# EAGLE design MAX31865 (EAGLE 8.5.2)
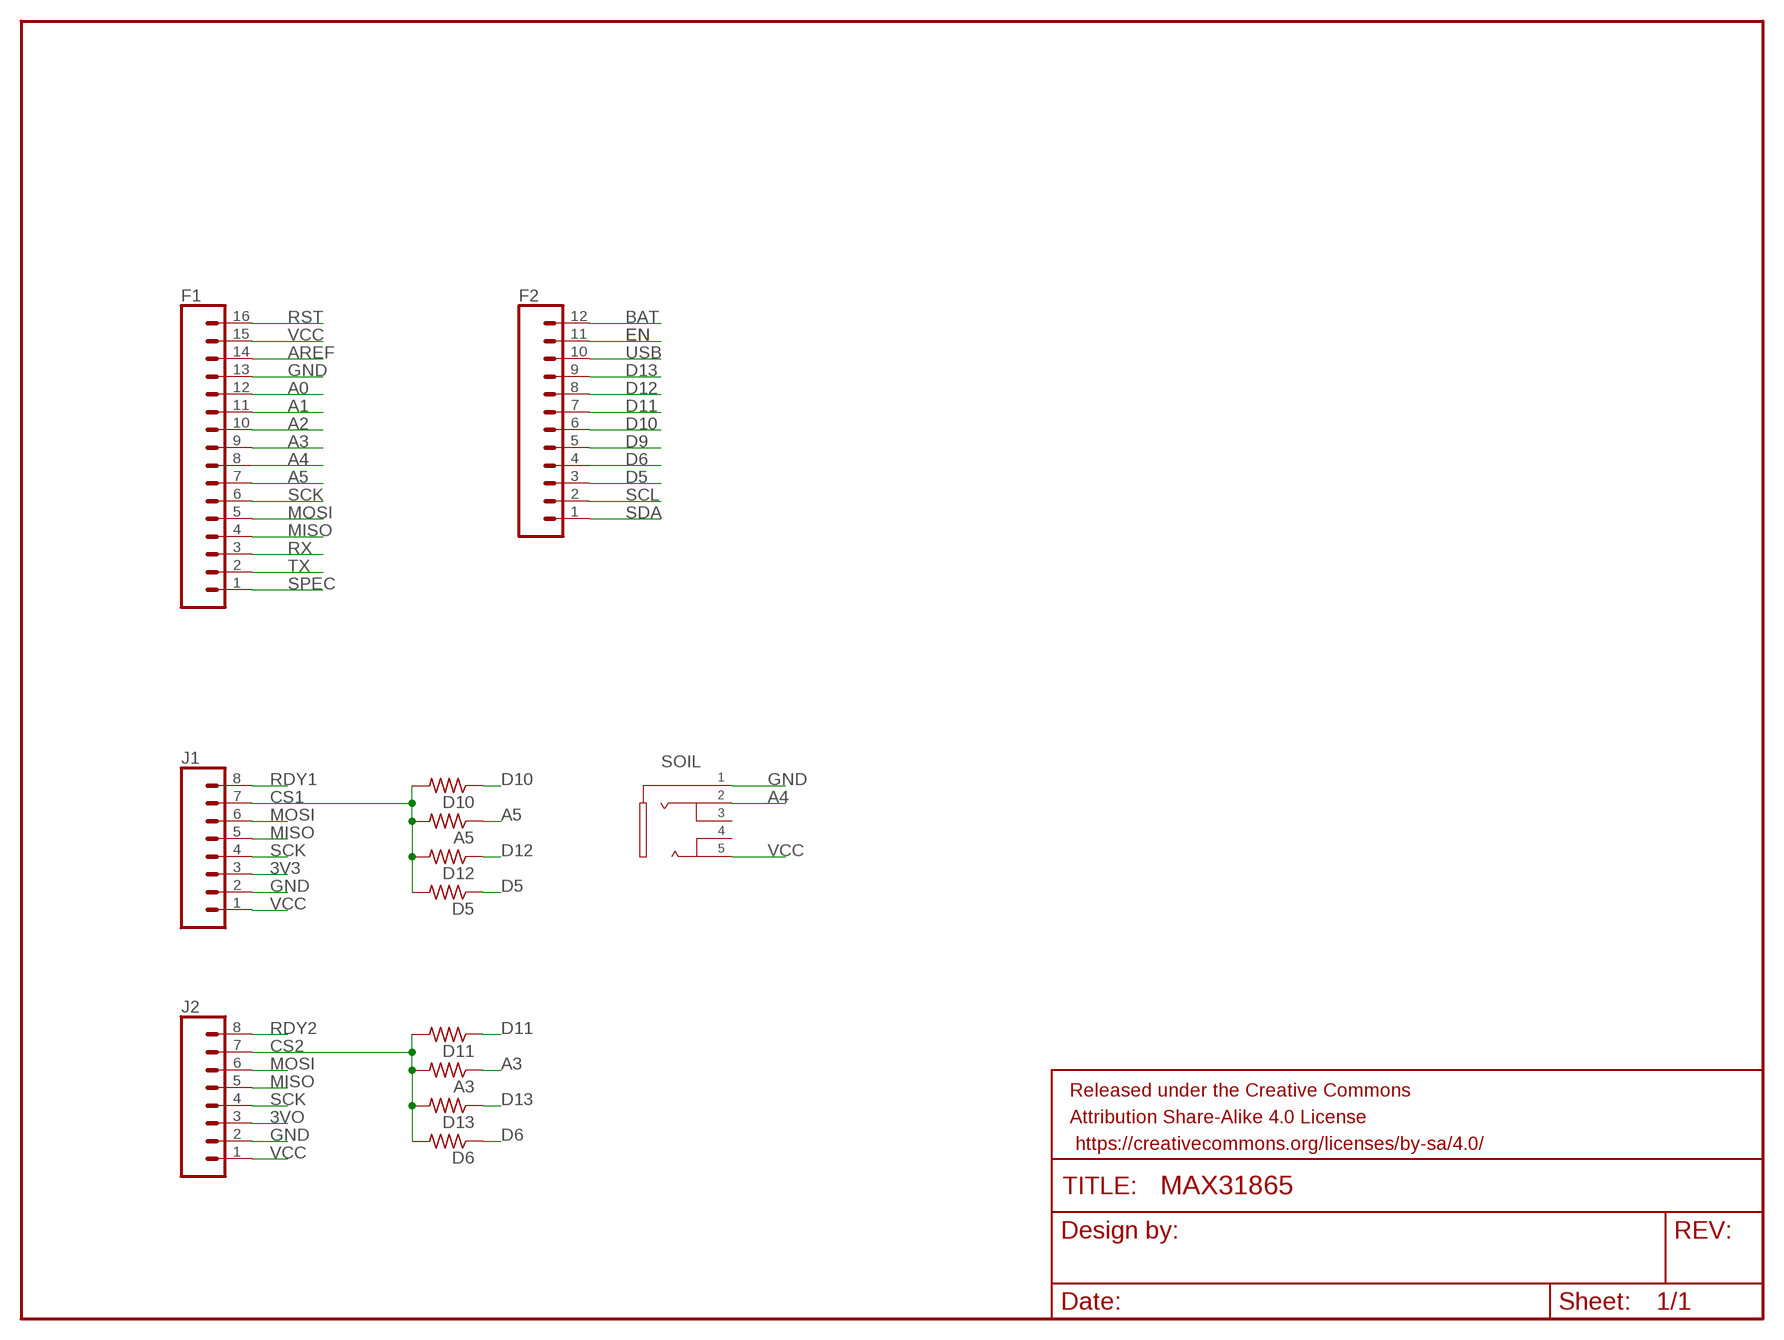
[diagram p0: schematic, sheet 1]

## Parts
A3  R-US_R0603  [R0603]
A5  R-US_R0603  [R0603]
D5  R-US_R0603  [R0603]
D6  R-US_R0603  [R0603]
D10  R-US_R0603  [R0603]
D11  R-US_R0603  [R0603]
D12  R-US_R0603  [R0603]
D13  R-US_R0603  [R0603]
F1  CONN_16  [1X16]
F2  CONN_12  [1X12]
FRAME1  FRAME-LETTER  [CREATIVE_COMMONS]
J1  CONN_08"  [1X08]
J2  CONN_08"  [1X08]
SOIL  JW-PJ-307-5H  [JW-PJ-307-5H]

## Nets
3V3: J1.3
3VO: J2.3
A0: F1.12
A1: F1.11
A2: F1.10
A3: A3.1 F1.9
A4: F1.8 SOIL.2
A5: A5.1 F1.7
AREF: F1.14
BAT: F2.12
CS1: A5.2 D5.2 D10.2 D12.2 J1.7
CS2: A3.2 D6.2 D11.2 D13.2 J2.7
D5: D5.1 F2.3
D6: D6.1 F2.4
D9: F2.5
D10: D10.1 F2.6
D11: D11.1 F2.7
D12: D12.1 F2.8
D13: D13.1 F2.9
EN: F2.11
GND: F1.13 J1.2 J2.2 SOIL.1
MISO: F1.4 J1.5 J2.5
MOSI: F1.5 J1.6 J2.6
RDY1: J1.8
RDY2: J2.8
RST: F1.16
RX: F1.3
SCK: F1.6 J1.4 J2.4
SCL: F2.2
SDA: F2.1
SPEC: F1.1
TX: F1.2
USB: F2.10
VCC: F1.15 J1.1 J2.1 SOIL.5
Unconnected: SOIL.3 SOIL.4

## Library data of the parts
A3 A5 D5 D6 D10-D13 = rcl:R-US_: RESISTOR, American symbol; SPICEPREFIX: R
F1 = SparkFun-Connectors:CONN_16: Multi connection point. Often used as Generic Header-pin footprint for 0.1 inch spaced/style header connections On any of the 0.1 inch spaced packages, you can populate with these: Break Away Headers - Straight (PRT-00116) Break Away Male Headers - Right Angle (PRT-00553) Female Headers (PRT-00115)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
F2 = SparkFun-Connectors:CONN_12: Multi connection point. Often used as Generic Header-pin footprint for 0.1 inch spaced/style header connections On any of the 0.1 inch spaced packages, you can populate with these: Break Away Headers - Straight (PRT-00116) Break Away Male Headers - Right Angle (PRT-00553) Female Headers (PRT-00115)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
FRAME1 = SparkFun-Aesthetics:FRAME-LETTER: Schematic Frame - Letter
J1 J2 = SparkFun-Connectors:CONN_08: Multi connection point. Often used as Generic Header-pin footprint for 0.1 inch spaced/style header connections On any of the 0.1 inch spaced packages, you can populate with these: Break Away Headers - Straight (PRT-00116) Break Away Male Headers - Right Angle (PRT-00553) Female Headers (PRT-00115)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; PROD_ID: CONN-08438
SOIL = jack:JW-PJ-307-5

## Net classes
0 default: width 0.254 mm, clearance 0.205 mm
1 GND: width 0.61 mm

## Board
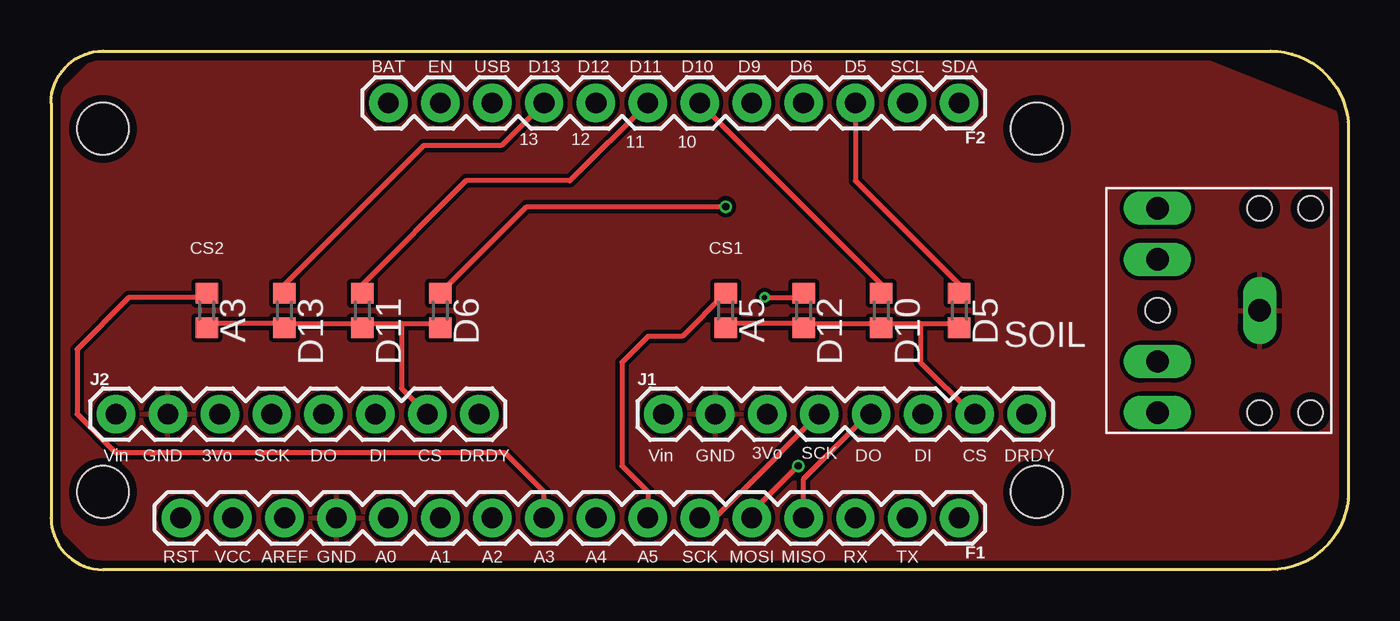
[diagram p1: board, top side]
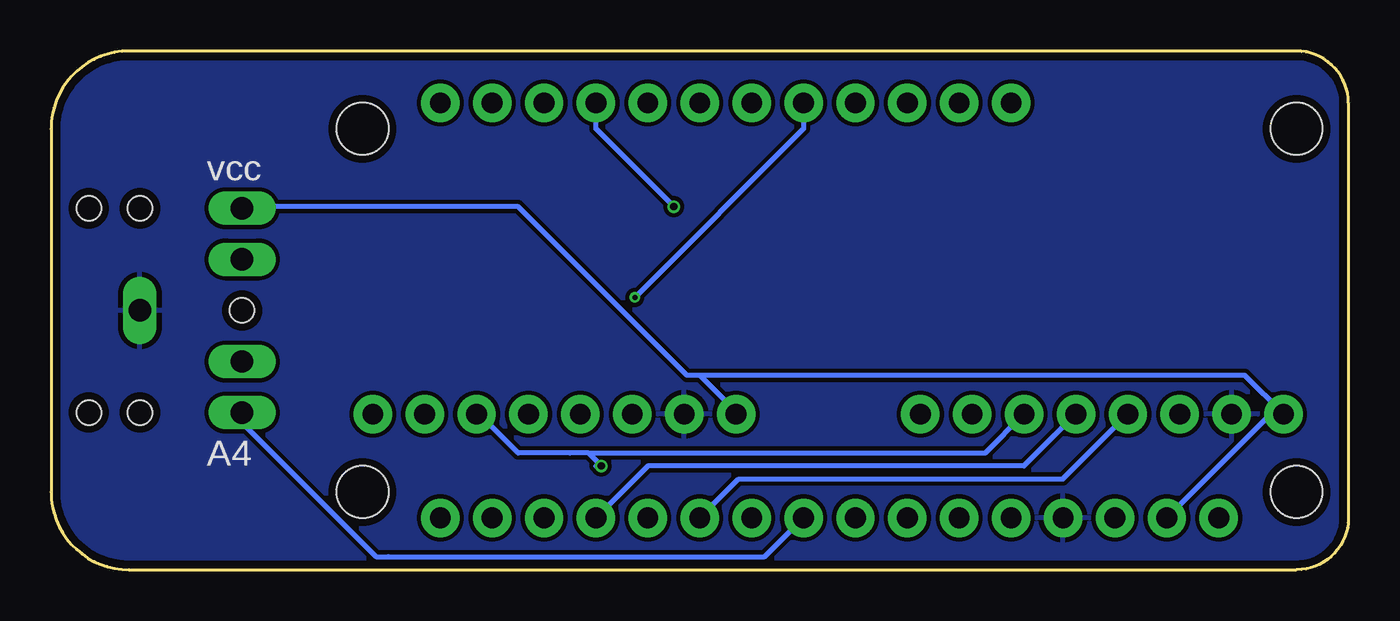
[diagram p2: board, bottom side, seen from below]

Size 63.5 x 25.4 mm. Coordinates in mm from the lower left corner, seen from the top.
Outline: 0,22.86 0,2.54 arc90 2.54,0 59.69,0 arc90 63.5,3.81 63.5,21.59 arc90 59.69,25.4 2.54,25.4 arc90 0,22.86
Copper layers (1*16): Top 0.035559375mm / dielectric 1.6mm / Bottom 0.035559375mm
Design rules "oshpark-2layer": minimum track width 6mil, minimum drill 10mil, track to track 6mil, track to pad 6mil, pad to pad 6mil, via to via 6mil, smd to smd 6mil, copper to edge 15mil, drill to drill 6mil, minimum pad ring 5mil, minimum via ring 5mil, stop-mask expansion 2.5mil, vias tented up to drill 0mil, thermal gap 10mil
Holes 2.54 mm at 48.26,3.81 48.26,21.59 2.54,3.81 2.54,21.59

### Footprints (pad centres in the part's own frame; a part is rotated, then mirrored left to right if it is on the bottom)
R0603 = smd 1 x 1.1: 1 -0.85,0; 2 0.85,0
1X16 = drill 1.016 pad 1.88: 1 0,0; 2 2.54,0; 3 5.08,0; 4 7.62,0; 5 10.16,0; 6 12.7,0; 7 15.24,0; 8 17.78,0; 9 20.32,0; 10 22.86,0; 11 25.4,0; 12 27.94,0; 13 30.48,0; 14 33.02,0; 15 35.56,0; 16 38.1,0
1X12 = drill 1.016 pad 1.88: 1 0,0; 2 2.54,0; 3 5.08,0; 4 7.62,0; 5 10.16,0; 6 12.7,0; 7 15.24,0; 8 17.78,0; 9 20.32,0; 10 22.86,0; 11 25.4,0; 12 27.94,0
1X08 = drill 1.016 pad 1.88: 1 0,0; 2 2.54,0; 3 5.08,0; 4 7.62,0; 5 10.16,0; 6 12.7,0; 7 15.24,0; 8 17.78,0
JW-PJ-307-5H = drill 1.1 long: 1 -2,0; 2 3,5; 3 3,2.5; 4 3,-2.5; 5 3,-5 | hole 1.2: -4.5,5; -2,5; 3,0; -4.5,-5; -2,-5

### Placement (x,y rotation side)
A3  7.62,12.7 270 top
A5  33.02,12.7 270 top
D5  44.45,12.7 270 top
D6  19.05,12.7 270 top
D10  40.64,12.7 270 top
D11  15.24,12.7 270 top
D12  36.83,12.7 270 top
D13  11.43,12.7 270 top
F1  44.45,2.54 180 top
F2  44.45,22.86 180 top
FRAME1  not placed on the board
J1  29.97,7.62 0 top
J2  3.17,7.62 0 top
SOIL  57.15,12.7 180 top

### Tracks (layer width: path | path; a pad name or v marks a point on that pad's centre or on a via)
A3
  Top 0.254: F1.9 24.13,3.81 22.22,5.71 3.17,5.71 1.27,7.62 1.27,10.79 3.81,13.34 7.41,13.34 A3.1
A4
  Bottom 0.254: SOIL.2 54.15,7.19 47.6,0.64 46.99,0.64 28.58,0.64 F1.8
A5
  Top 0.254: F1.7 29.21,3.81 27.94,5.08 27.94,10.16 29.21,11.43 30.9,11.43 A5.1
CS1
  Top 0.254: 36.83,12.06 33.02,12.06 A5.2 | 36.83,12.06 40.64,12.06 | 36.83,12.06 D12.2 | 40.64,12.06 42.55,12.06 | 42.55,12.06 44.45,12.06 D5.2 | 40.64,12.06 D10.2 | 42.55,12.06 42.55,10.16 45.09,7.62 J1.7
CS2
  Top 0.254: 11.43,12.06 7.62,12.06 A3.2 | 11.43,12.06 15.24,12.06 | 11.43,12.06 D13.2 | 15.24,12.06 17.14,12.06 | 17.14,12.06 19.05,12.06 D6.2 | 15.24,12.06 D11.2 | J2.7 17.14,8.89 17.14,12.06
D5
  Top 0.254: F2.3 39.37,19.05 44.45,13.97 D5.1
D6  (via drill 0.35)
  Top 0.254: D6.1 23.28,17.78 v33.02,17.78
  Bottom 0.254: v33.02,17.78 36.83,21.59 F2.4
D10
  Top 0.254: F2.6 31.75,22.23 32.38,22.23 40.64,13.97 D10.1
D11
  Top 0.254: D11.1 15.24,13.97 20.32,19.05 25.4,19.05 F2.7
D12  (via drill 0.25)
  Top 0.254: v34.92,13.34 36.83,13.34 D12.1
  Bottom 0.254: v34.92,13.34 26.67,21.59 F2.8
D13
  Top 0.254: D13.1 11.43,13.97 18.24,20.78 22.05,20.78 F2.9
GND
  pour Top: 0,22.86 0,2.54 2.54,0 50.8,-0.25 63.5,-0.25 64.77,21.59 52.07,26.67 2.54,25.4
  pour Bottom: 0,25.4 0,0 74.93,0 63.5,26.67
MISO
  Top 0.254: F1.4 36.83,4.45 40.01,7.62 J1.5
  Bottom 0.254: J2.5 15.88,5.08 34.29,5.08 F1.4
MOSI  (via drill 0.35)
  Top 0.254: v36.57,5.08 34.29,2.8 F1.5
  Bottom 0.254: J2.6 17.78,5.71 37.2,5.71 | J1.6 42.55,7.62 40.64,5.71 38.1,5.71 37.2,5.71 | 36.83,5.08 v36.57,5.08 37.2,5.71
SCK
  Top 0.254: J1.4 33.78,3.81 33.76,3.81 32.49,2.54 F1.6
  Bottom 0.254: J2.4 13.97,4.45 29.84,4.45 31.12,3.17 31.12,2.54 F1.6
VCC
  Bottom 0.254: 31.75,9.53 32.38,9.53 40.64,17.78 53.98,17.78 SOIL.5 | 31.75,9.53 29.84,7.62 J1.1 | 31.75,9.53 5.08,9.53 J2.1 3.81,7.62 F1.15

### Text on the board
tPlace: BAT | EN | USB | D13 | D12 | D11 | D10 | D9 | D6 | D5 | SCL | SDA | 13 | 12 | 11 | 10 | CS2 | CS1 | Vin | GND | 3Vo | SCK | DO | DI | CS | DRDY | Vin | GND | 3Vo | SCK | DO | DI | CS | DRDY | RST | VCC | AREF | GND | A0 | A1 | A2 | A3 | A4 | A5 | SCK | MOSI | MISO | RX | TX
bNames: vcc | A4

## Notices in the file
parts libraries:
SparkFun-Connectors: Licensing: Creative Commons ShareAlike 4.0 International - https://creativecommons.org/licenses/by-sa/4.0
SparkFun-Aesthetics: Released under the Creative Commons Attribution Share-Alike 4.0 License
SparkFun-Aesthetics: https://creativecommons.org/licenses/by-sa/4.0
